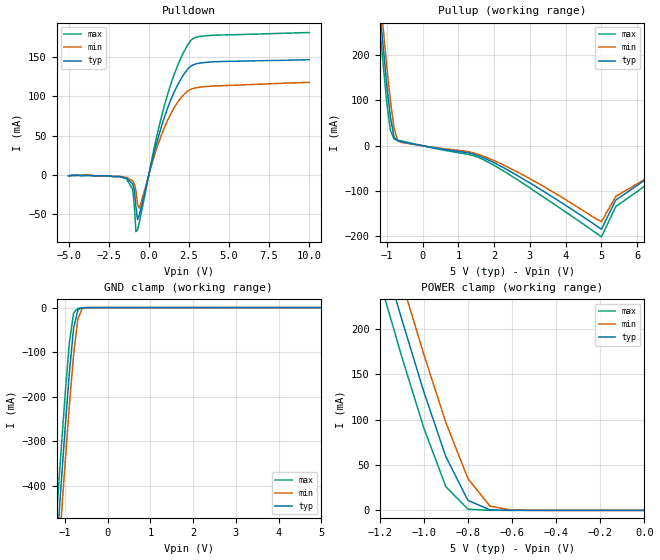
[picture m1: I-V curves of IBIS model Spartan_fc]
|   * spartan_fc.ibs * IBIS 1.1 Model for Spartan
[IBIS Ver]	1.1
[Comment char]	|_char
[File name]	spartan_fc.ibs
[Date]		Fri Jan 23 16:10:30 1998
[File Rev]	1.0
[Source] s2ibis Version 1.0 SPICE to IBIS converter
   s05-1e.lib, s05-1ediode.mod
[Notes]   Spartan 5V process
[Disclaimer]
The data in this model is derived from SPICE simulations using modeling
information extracted from the target process.  While a great deal of
care has been taken to provide information that is accurate, this model
is considered preliminary as it has not been verified by actual silicon
measurement.  Treat the data in this model as preliminary until actual
silicon verification is performed.
| Spartan - Fast, CMOS
|   COMPONENT: Spartan
[Component]	Spartan
[Manufacturer]	Xilinx
[Package]
| Note: approximate package data for PQ's
|   typ   min   max
R_pkg   60m   40m   80m
L_pkg   13nH   10nH   16nH
C_pkg   1.4pF   0.7pF   2pF
[Pin] signal_name model_name R_pin L_pin C_pin
all   iob   Spartan_fc
2 GND GND
3 VDD POWER
| Models and submodels in the file (1): Spartan_fc (I/O)
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|   MODEL Spartan_fc
[Model]		Spartan_fc
Model_type	I/O
Polarity	Non-Inverting
Enable		Active-Low
Vinh  = 2.0V
Vinl  = 0.8V
C_comp   7.0p   5.0p   9.0p
[Voltage range]   5.000   4.500   5.500
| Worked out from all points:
|   slope of the pulldown table from 0 to 0.75 V, typ, clamps not added: 12.8 ohm
|   slope of the pullup table from 0 to 0.75 V, typ, clamps not added: 77.1 ohm
|   GND clamp passes 1 mA (typ) near -0.61 V on its own axis
|   POWER clamp passes 1 mA (typ) near -0.70 V on its own axis
[Pulldown]
|  Voltage   I(typ)   I(min)   I(max)
-5V       -1mA       -1mA       -1mA
-1.4V     -3.9mA     -3.1mA     -4.7mA
-1V       -11.3mA    -7.5mA     -18.3mA
-900mV    -19.4mA    -11.3mA    -39.37mA
-800mV    -40.4mA    -19.7mA    -71.92mA
-700mV    -56.79mA   -37mA      -69.71mA
-600mV    -51.51mA   -42.23mA   -60.92mA
400mV     33.53mA    27.75mA    40.02mA
1.1V      80.62mA    65.99mA    97.02mA
1.9V      118mA      95.03mA    143.8mA
2.6V      137.7mA    108.5mA    170.3mA
10V       146.2mA    117.6mA    180.7mA
[GND_clamp]
|  Voltage   I(typ)   I(min)   I(max)
-5V       -6.234A    -6.302A    -6.168A
-1.2V     -547.5mA   -626.3mA   -469.9mA
-1.1V     -407.8mA   -486.4mA   -330.4mA
-1V       -272.7mA   -350.3mA   -197.1mA
-900mV    -147.2mA   -220.8mA   -79.43mA
-800mV    -46.44mA   -105.5mA   -11.87mA
-700mV    -5.189mA   -25.6mA    -1.885mA
-600mV    -708.8uA   -2.512mA   -491.3uA
-500mV    -139.3uA   -303.7uA   -65.15uA
5V        150.7pA    16.26uA    111.2pA
[Pullup]
|  Voltage   I(typ)   I(min)   I(max)
-5V       3.726A     3.76A      3.696A
-1.4V     466.8mA    508.1mA    426.5mA
-1V       132.8mA    173.2mA    94.07mA
-900mV    63.02mA    99.04mA    33.79mA
-800mV    19.54mA    39.5mA     14.95mA
-700mV    10.72mA    12.14mA    12.52mA
-600mV    8.899mA    7.607mA    10.73mA
1.7V      -26.51mA   -23.02mA   -30.79mA
3V        -82.06mA   -72.69mA   -93.08mA
5V        -184mA     -167.4mA   -200.8mA
5.4V      -119.6mA   -111.6mA   -134.1mA
10V       127.9mA    101.9mA    121.6mA
[POWER_clamp]
|  Voltage   I(typ)   I(min)   I(max)
-5V       3.726A     3.76A      3.696A
-1.2V     293.8mA    335.7mA    252.7mA
-1.1V     210.3mA    252.2mA    169.3mA
-1V       130.6mA    171.7mA    90.75mA
-900mV    59.07mA    96.7mA     26.03mA
-800mV    10.99mA    35.01mA    1.277mA
-700mV    516uA      4.619mA    24.5uA
-600mV    18.72uA    277.8uA    467.8nA
0V        150.7pA    780.8pA    133.6pA
[Ramp]
|  variable   typ   min   max
dV/dt_r   1.58/0.64n   1.32/0.81n   1.86/0.51n
dV/dt_f   2.36/0.72n   2.02/0.90n   2.70/0.60n
